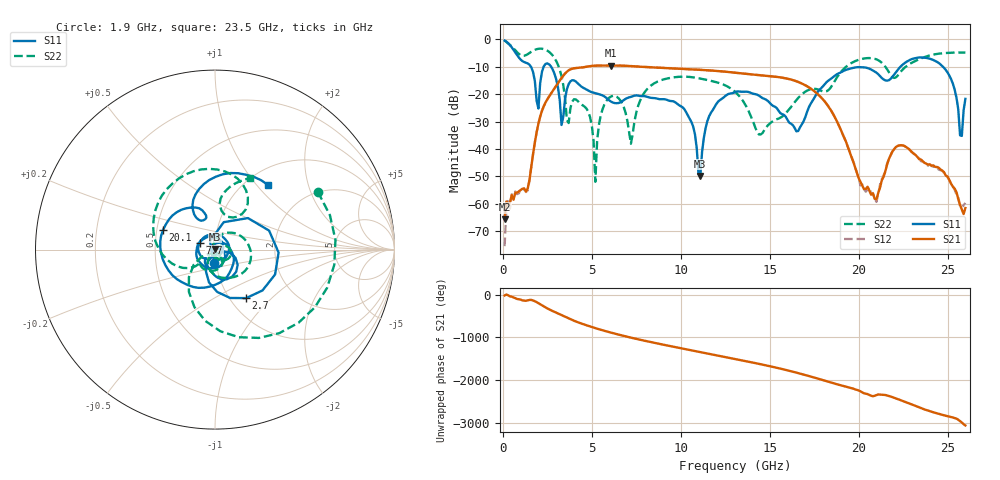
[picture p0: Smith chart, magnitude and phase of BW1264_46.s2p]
!Keysight Technologies,N5245B,MY57181159,A.13.60.06
!Date: Friday, December 18, 2020 23:54:30
!Correction: S11(Full 2 Port(1,2))
!S21(Full 2 Port(1,2))
!S12(Full 2 Port(1,2))
!S22(Full 2 Port(1,2))
!S2P File: Measurements: S11, S21, S12, S22:
# Hz S  dB  R 50
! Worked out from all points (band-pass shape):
!   260 points, 100 MHz to 26 GHz, reference 50 ohm
!   highest |S21| = -9.59 dB at 6.1 GHz (marker M1); lowest = -65.6 dB at 100 MHz (marker M2)
!   |S21| within 3 dB of the highest: 3.488 GHz to 13.63 GHz (10.14 GHz wide, 118 % of centre)
!   lowest |S11| = -49.8 dB at 11.1 GHz (marker M3), VSWR 1.01, Z = 50.1 + j0.298 ohm
!   |S11| at or under -10 dB: 1.574 GHz to 2.295 GHz (720.9 MHz wide, 37.3 % of centre); 2.712 GHz to 22.36 GHz (19.64 GHz wide, 157 % of centre); 24.73 GHz to end of sweep
!   |S22| runs from -52.0 to -0.5 dB; largest |S21 - S12| = 0.00066
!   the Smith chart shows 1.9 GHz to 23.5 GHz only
!   S11 on the Smith chart (normalised r, x): 1.9 GHz: 0.98, -0.15; 2.7 GHz: 1.19, -0.71; 7.7 GHz: 0.84, +0.06; 20.1 GHz: 0.54, +0.13; 23.5 GHz: 1.25, +1.15
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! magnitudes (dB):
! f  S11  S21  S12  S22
! 100 MHz  -0.5  -65.6  -75.4  -0.5
! 1.9 GHz  -22.4  -33.9  -33.9  -3.6
! 2.7 GHz  -9.9  -19.9  -19.9  -5.2
! 3.3 GHz  -31.3  -14.1  -14.1  -13.5
! 4.5 GHz  -17.6  -10.3  -10.3  -24.2
! 5.2 GHz  -19.7  -9.6  -9.6  -52.0
! 5.4 GHz  -20.0  -9.6  -9.6  -31.2
! 6.1 GHz  -22.8  -9.6  -9.6  -20.8
! 7.2 GHz  -21.0  -9.8  -9.8  -38.1
! 7.7 GHz  -20.7  -10.0  -10.0  -22.6
! 8.8 GHz  -21.8  -10.4  -10.4  -15.2
! 11.1 GHz  -49.8  -11.2  -11.2  -14.3
! 11.6 GHz  -28.0  -11.4  -11.4  -15.0
! 13.1 GHz  -19.2  -12.2  -12.2  -19.4
! 14.4 GHz  -20.6  -13.1  -13.1  -34.7
! 17.4 GHz  -22.5  -18.4  -18.4  -18.1
! 20.1 GHz  -10.2  -51.9  -53.3  -7.3
! 21.7 GHz  -14.9  -43.6  -43.7  -12.0
! 23.5 GHz  -6.6  -43.8  -44.4  -7.0
! 25.1 GHz  -13.3  -51.3  -51.3  -5.0
! 25.7 GHz  -35.0  -60.4  -61.0  -4.9
! 26 GHz  -21.7  -61.5  -59.6  -4.9
